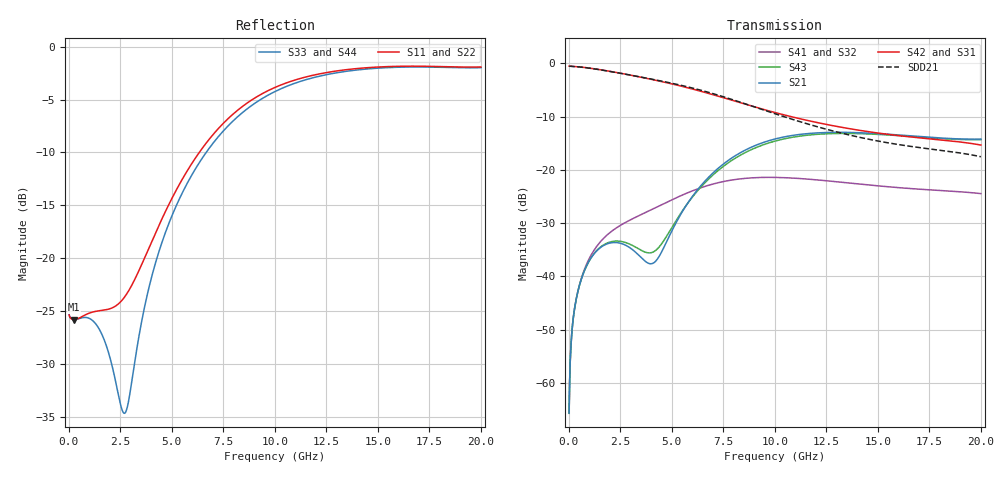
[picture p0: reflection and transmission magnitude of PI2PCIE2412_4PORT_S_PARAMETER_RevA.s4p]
! NPort=4 DATA=800 NOISE=0 GROUPDELAY=0 COMPLEX_DATAFORMAT=POLAR
! NumOfBlock=1 NumOfParam=0
! .MODEL Smodel S TSTONEFILE=PI2PCIE2412_4PORT_S_PARAMETER_RevA.s4p TYPE=S
!  -- The above .MODEL line can be used for the S element in the netlist.
! PORT DEFINITION
! PORT1 = INPUT+
! PORT2 = INPUT-
! PORT3 = OUTPUT+
! PORT4 = OUTPUT-
# Hz S MA R  50
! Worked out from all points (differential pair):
!   800 points, 25 MHz to 20 GHz, reference 50 ohm
!   strongest paths, dB at 25 MHz, 5.025 GHz, 10.03 GHz, 15.03 GHz, 20 GHz:
!     S42: -0.5, -3.9, -9.3, -13.1, -15.4
!     S31: -0.5, -3.9, -9.3, -13.1, -15.4
!     S21: -65.7, -31.4, -14.2, -13.2, -14.2
!     S43: -65.7, -30.7, -14.6, -13.4, -14.3
!     S41: -65.7, -25.6, -21.4, -23.0, -24.5
!     S32: -65.7, -25.6, -21.4, -23.0, -24.5
!   taken as a pair (ports 2,1 in; 4,3 out), SDD21 dB: -0.5, -3.8, -9.5, -14.6, -17.5
!   lowest |S11| = -25.8 dB at 275 MHz (marker M1), VSWR 1.11, Z = 55.2 - j1.32 ohm
!   |S11| at or under -10 dB: start of sweep to 6.337 GHz
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2.5e7  0.05402 -3.0  0.0005195 87.5  0.9399 -0.7  0.0005171 87.4
       0.0005195 87.5  0.05402 -3.0  0.0005171 87.4  0.9399 -0.7
       0.9399 -0.7  0.0005171 87.4  0.05411 -2.4  0.0005196 87.5
       0.0005171 87.4  0.9399 -0.7  0.0005196 87.5  0.05411 -2.4
2.75e8  0.05136 -13.4  0.004775 74.9  0.9333 -6.1  0.004773 74.4
        0.004775 74.9  0.05136 -13.4  0.004773 74.4  0.9333 -6.1
        0.9333 -6.1  0.004773 74.4  0.05131 -7.0  0.004774 75.2
        0.004773 74.4  0.9333 -6.1  0.004774 75.2  0.05131 -7.0
2.75e9  0.06643 -168.2  0.01965 44.6  0.7915 -53.3  0.03197 34.1
        0.01965 44.6  0.06643 -168.2  0.03197 34.1  0.7915 -53.3
        0.7914 -53.4  0.03196 34.1  0.01869 -164.7  0.0208 48.9
        0.03196 34.1  0.7914 -53.4  0.0208 48.9  0.01869 -164.7
4.175e9  0.1291 111.2  0.01358 88.9  0.6962 -77.0  0.04373 17.9
         0.01358 88.9  0.1291 111.2  0.04373 17.9  0.6962 -77.0
         0.6961 -77.0  0.04373 17.9  0.09221 85.2  0.01723 84.4
         0.04373 17.9  0.6961 -77.0  0.01723 84.4  0.09221 85.2
7.55e9  0.4386 13.2  0.1149 104.6  0.4727 -126.7  0.07789 -34.2
        0.1149 104.6  0.4386 13.2  0.07789 -34.2  0.4727 -126.7
        0.4726 -126.7  0.07787 -34.2  0.4039 6.5  0.1093 100.5
        0.07787 -34.2  0.4726 -126.7  0.1093 100.5  0.4039 6.5
1.31e10  0.7696 -66.3  0.2248 33.5  0.2537 176.0  0.07694 -124.7
         0.2248 33.5  0.7696 -66.3  0.07694 -124.7  0.2537 176.0
         0.2536 175.9  0.07691 -124.7  0.7548 -67.1  0.2194 33.6
         0.07691 -124.7  0.2536 175.9  0.2194 33.6  0.7548 -67.1
2e10  0.8013 -102.8  0.1942 0.5  0.1709 97.9  0.0598 140.1
      0.1942 0.5  0.8013 -102.8  0.0598 140.1  0.1709 97.9
      0.1708 97.9  0.05976 140.0  0.7951 -103.0  0.1922 0.9
      0.05976 140.0  0.1708 97.9  0.1922 0.9  0.7951 -103.0
